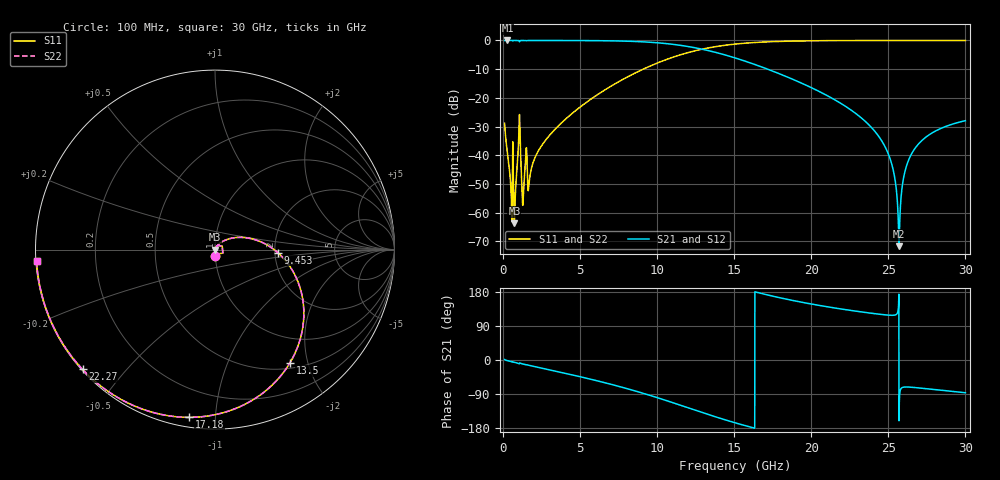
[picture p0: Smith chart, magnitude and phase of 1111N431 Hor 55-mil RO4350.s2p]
# GHz S MA R 50
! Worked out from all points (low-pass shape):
!   3201 points, 100 MHz to 30 GHz, reference 50 ohm
!   highest |S21| = 0.00 dB at 286.9 MHz (marker M1); lowest = -71.7 dB at 25.69 GHz (marker M2)
!   |S21| within 3 dB of the highest: start of sweep to 12.88 GHz
!   lowest |S11| = -63.7 dB at 735.4 MHz (marker M3), VSWR 1.00, Z = 50.1 - j0.00042 ohm
!   |S11| at or under -10 dB: start of sweep to 9.092 GHz
!   |S22| runs from -63.7 to 0.0 dB; largest |S21 - S12| = 0
!   S11 on the Smith chart (normalised r, x): 100 MHz: 1.00, -0.07; 9.453 GHz: 2.07, -0.08; 13.5 GHz: 0.58, -1.71; 17.18 GHz: 0.05, -0.86; 22.27 GHz: 0.00, -0.38; 30 GHz: 0.00, -0.03
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0.1  0.03613 -88.4  0.9991 1.2  0.9991 1.2  0.03613 -88.4
0.286875  0.01068 -89.9  0.9996 -1.8  0.9996 -1.8  0.01068 -89.9
0.62325  0.01044 38.9  0.9924 -5.6  0.9924 -5.6  0.01044 38.9
0.735375  0.0006511 -0.4  0.9993 -6.1  0.9993 -6.1  0.0006511 -0.4
0.8381563  0.003345 70.1  0.9992 -7.1  0.9992 -7.1  0.003345 70.1
1.025031  0.02365 57.7  0.9906 -9.7  0.9906 -9.7  0.02365 57.7
1.314688  0.001934 37.7  0.9986 -10.9  0.9986 -10.9  0.001934 37.7
2.71625  0.01771 63.8  0.9986 -23.2  0.9986 -23.2  0.01771 63.8
5.089563  0.07219 44.1  0.9956 -44.9  0.9956 -44.9  0.07219 44.1
9.453094  0.3497 -2.7  0.9334 -92.3  0.9334 -92.3  0.3497 -2.7
10.06978  0.4106 -10.5  0.908 -100.2  0.908 -100.2  0.4106 -10.5
13.49894  0.7564 -56.5  0.6483 -146.2  0.6483 -146.2  0.7564 -56.5
15.05  0.8638 -75.9  0.4967 -165.6  0.4967 -165.6  0.8638 -75.9
17.18038  0.9458 -98.8  0.315 171.5  0.315 171.5  0.9458 -98.8
20.03956  0.9861 -122.9  0.149 147.4  0.149 147.4  0.9861 -122.9
22.27272  0.995 -137.9  0.06973 132.6  0.06973 132.6  0.995 -137.9
25.01978  0.9974 -153.4  0.01021 118.3  0.01021 118.3  0.9974 -153.4
25.37484  0.9974 -155.2  0.004665 118.3  0.004665 118.3  0.9974 -155.2
25.69253  0.9974 -156.8  0.0002611 -160.4  0.0002611 -160.4  0.9974 -156.8
26.09431  0.9974 -158.8  0.005441 -71.3  0.005441 -71.3  0.9974 -158.8
26.73903  0.9973 -161.9  0.0133 -72.8  0.0133 -72.8  0.9973 -161.9
30  0.9965 -176.3  0.04007 -86.4  0.04007 -86.4  0.9965 -176.3
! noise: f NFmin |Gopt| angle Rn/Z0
0.1  0.0006681  0.7352  0.9257  0.000504
3.417  0.008371  0.4215  27.15  0.002259
6.743  0.0149  0.4011  49.28  0.003443
10.06  0.02357  0.4593  67.29  0.005385
13.39  0.03811  0.5785  85.01  0.009467
16.7  0.06829  0.7306  104.9  0.01955
20.03  0.149  0.8667  125.6  0.05124
23.35  0.5128  0.9588  144.7  0.2601
26.67  1.768  0.9873  161.5  0.8445
30  0.5859  0.9605  176.3  0.004955
